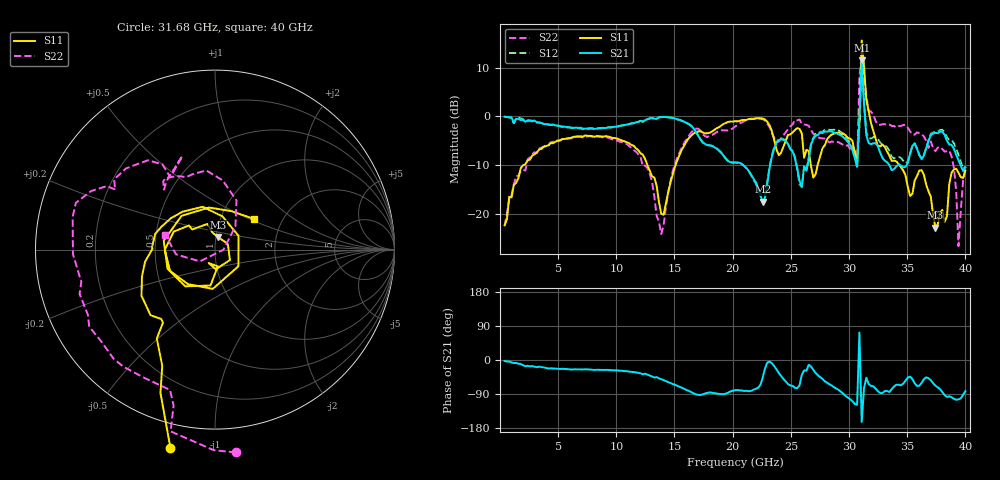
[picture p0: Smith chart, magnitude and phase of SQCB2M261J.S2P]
! Network Analyzer HP8722ES.07.66: Jul 25, 2000 Serial No. US39175408
! 27 Oct 2004  13:56:13
! Frequency  S11  S21  S12  S22
# HZ  S  DB R  50
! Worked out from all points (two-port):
!   201 points, 400 MHz to 40 GHz, reference 50 ohm
!   highest |S21| = 11.52 dB at 31.09 GHz (marker M1); lowest = -17.5 dB at 22.58 GHz (marker M2)
!   |S21| within 3 dB of the highest: 31.03941 GHz to 31.15571 GHz (116.3 MHz wide, 0.374 % of centre)
!   lowest |S11| = -22.8 dB at 37.43 GHz (marker M3), VSWR 1.16, Z = 51 + j7.23 ohm
!   |S11| at or under -10 dB: start of sweep to 2.037 GHz; 12.67 GHz to 15.1 GHz (2.431 GHz wide, 17.5 % of centre); 34.33 GHz to end of sweep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
!   |S22| runs from -26.6 to 12.4 dB; largest |S21 - S12| = 0.46
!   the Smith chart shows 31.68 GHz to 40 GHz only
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4e8  -22.36 -100.6  -0.10 -2.7  -0.07 -2.2  -22.46 -97.8
7.132e9  -4.19 -108.2  -2.55 -25.0  -2.65 -26.0  -4.38 -119.3
1.1686e10  -6.56 -107.9  -1.23 -32.8  -1.23 -33.1  -7.24 -134.4
1.3666e10  -17.60 -93.4  -0.23 -48.3  -0.19 -48.3  -21.62 176.8
1.6438e10  -3.95 3.9  -1.95 -85.1  -1.98 -85.3  -3.31 3.7
2.02e10  -1.01 1.9  -9.45 -79.7  -9.51 -79.7  -2.12 -7.9
2.2576e10  -0.45 -14.5  -17.52 -47.2  -17.66 -43.8  -0.58 -23.8
2.3962e10  -8.00 -14.4  -4.90 -34.3  -4.68 -33.8  -5.21 -12.9
2.5546e10  -2.42 -15.9  -10.67 -74.3  -10.63 -76.0  -0.84 -9.3
2.6932e10  -12.59 -173.2  -4.61 -26.1  -4.42 -23.7  -3.61 -34.2
2.8318e10  -4.12 68.2  -3.05 -64.0  -2.80 -58.6  -5.37 -30.6
3.0694e10  -8.57 10.9  -10.40 -118.3  -9.87 -113.0  -10.69 -42.3
3.0892e10  -1.45 10.4  -0.22 72.4  -2.11 86.9  8.13 -25.4
3.109e10  15.55 -75.6  11.52 -163.6  11.80 -156.9  12.41 157.3
3.1288e10  10.30 -68.8  2.48 -74.1  3.06 -66.9  7.51 -93.5
3.1486e10  3.32 -76.9  -3.90 -46.7  -3.30 -41.6  4.28 -68.7
3.1684e10  1.10 -102.6  -5.49 -63.2  -4.48 -57.5  1.11 -84.1
3.3466e10  -8.05 -170.2  -9.99 -84.6  -7.09 -87.6  -1.70 -148.5
3.7426e10  -22.84 77.8  -3.41 -67.8  -3.09 -69.0  -7.16 130.3
3.8812e10  -11.59 -129.0  -5.87 -98.4  -4.79 -99.4  -8.23 83.6
3.9406e10  -11.54 134.7  -9.03 -103.8  -7.89 -108.5  -26.65 -1.4
4e10  -11.13 37.8  -10.48 -82.1  -10.32 -85.6  -10.79 163.5
